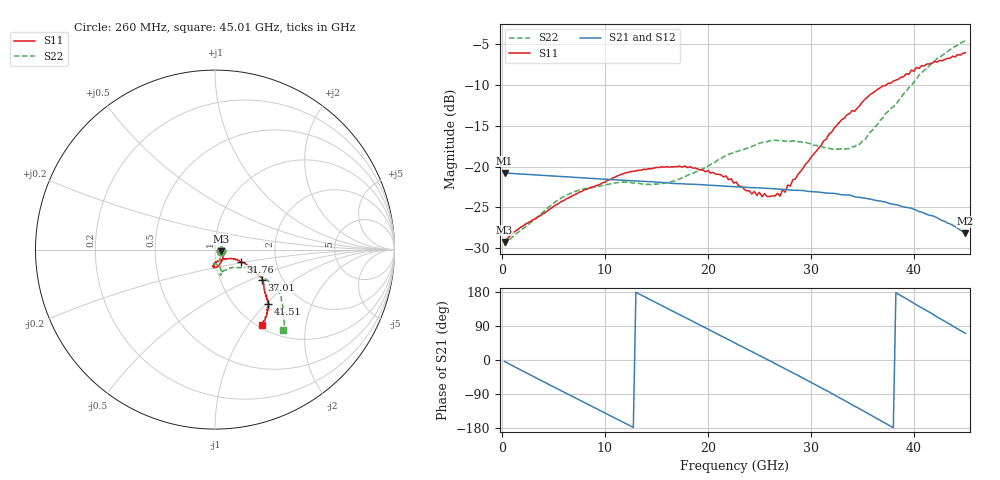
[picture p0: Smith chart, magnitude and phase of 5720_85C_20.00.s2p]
! Device:  ADRF5720
! Description: 0.5dB LSB GaAs MMIC 6-bit Digital Attenuator
! Frequency:  0.000009 -  40 GHz
! Ports:
!	RF1	= Port 1
!	RF2	= Port 2
! Vdd:  3.3 Volt
! Vss:  -3.3 Volt
! Control:  0/3.3 Volt
! State:  20.00 dB attenuation
! Data:  The device was measured using G-S-G Probes on a matrix board.
!  Data was collected using an calibrated 4 port network analyzer.
!  The reference plane for this measurement is at the launchers.
! Note:  Analog Devices supplies this data as a sample of measured data
!  for this product.  Your particular data for this product may vary.
!  Data was taken at 85 degrees C.
!  Analog Devices reserves the right to change this data at anytime.
# GHZ S DB R 45.0
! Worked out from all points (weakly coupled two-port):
!   180 points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, 260 MHz to 45.01 GHz, reference 45 ohm
!   highest |S21| = -20.79 dB at 260 MHz (marker M1); lowest = -28.1 dB at 45.01 GHz (marker M2)
!   lowest |S11| = -29.2 dB at 260 MHz (marker M3), VSWR 1.07, Z = 48.1 - j0.786 ohm
!   |S11| at or under -10 dB: start of sweep to 37.35 GHz
!   |S22| runs from -29.7 to -4.6 dB; largest |S21 - S12| = 0.00047
!   S11 on the Smith chart (normalised r, x): 260 MHz: 1.07, -0.02; 31.76 GHz: 1.32, -0.18; 37.01 GHz: 1.58, -0.58; 41.51 GHz: 1.39, -1.03; 45.01 GHz: 1.04, -1.16
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0.26  -29.23 -13.7  -20.79 -3.9  -20.78 -3.9  -29.73 -15.6
1.26  -27.93 -4.0  -20.88 -18.3  -20.87 -18.3  -28.34 -13.0
5.26  -24.68 -40.1  -21.18 -74.2  -21.16 -74.2  -24.26 -65.1
7.76  -23.04 -54.9  -21.37 -108.8  -21.36 -108.8  -22.80 -80.3
12.01  -20.76 -75.6  -21.69 -167.5  -21.68 -167.4  -21.90 -92.6
15.26  -20.12 -87.5  -21.91 147.3  -21.90 147.4  -22.12 -88.7
18.26  -20.02 -94.4  -22.15 105.9  -22.14 106.0  -20.95 -79.2
22.76  -21.89 -91.7  -22.48 43.3  -22.46 43.5  -18.18 -73.8
24.26  -23.35 -84.9  -22.59 22.5  -22.57 22.7  -17.55 -74.9
27.01  -23.60 -54.0  -22.75 -16.3  -22.73 -16.0  -16.86 -76.6
27.26  -22.82 -48.9  -22.79 -19.9  -22.78 -19.7  -16.84 -77.3
27.51  -23.15 -47.6  -22.82 -23.3  -22.81 -23.1  -16.93 -76.9
27.76  -22.27 -43.0  -22.84 -26.8  -22.83 -26.6  -16.82 -77.7
28.01  -22.39 -43.0  -22.88 -30.4  -22.86 -30.2  -16.92 -77.5
30.26  -18.52 -27.6  -23.07 -62.5  -23.06 -62.3  -17.43 -76.3
31.76  -16.03 -25.4  -23.25 -84.1  -23.24 -83.8  -17.79 -70.7
34.76  -12.53 -27.8  -23.77 -129.2  -23.76 -128.9  -17.27 -46.2
37.01  -10.15 -32.6  -24.30 -163.5  -24.28 -163.1  -14.07 -29.8
37.76  -9.82 -33.9  -24.56 -175.0  -24.54 -174.6  -12.91 -28.3
41.51  -7.46 -46.0  -25.96 126.2  -25.93 126.6  -7.69 -32.7
43.51  -6.78 -50.4  -27.01 94.4  -26.98 94.7  -5.71 -42.2
45.01  -6.09 -58.4  -28.14 70.4  -28.10 70.7  -4.60 -49.9
